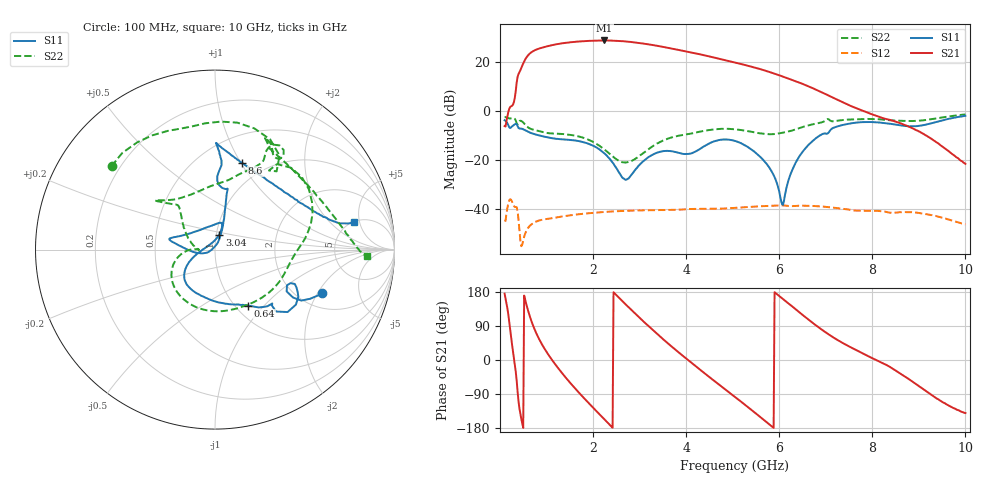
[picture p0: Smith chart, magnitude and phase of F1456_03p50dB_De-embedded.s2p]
! Integrated Device Technology
! Corporate Headquarters
! 6024 Silver Creek Valley Road
! San Jose, CA 95138  USA
! Phone:  1-408-284-8200
! Toll Free:  1-800-223-1366
! Webpage:  http://www.idt.com/
! Timing and RF Division
! 515 Groton Road, Suite 102
! Westford, MA 01886-6024
! Device:  F1456
! Description: 6-bit 0.5 dB Transmit Variable Gain Amplifier
! Frequency:  2100.0 -  2950.00 MHz
! Package:  6x6 mm Thin QFN Plastic Package: 28 pin
! State:  7
! Atten State:  3.5 dB
! Voltage:  +5.00 Volts
! Current:  214.736 mA
! Data:  The device was measured on a the F1455 evaluation board which has
!  individual transmission lines to the RF pins.  Data was collected
!  using a calibrated network analyzer.  The evaluation board was
!  de-embedded using a TRL calibration technique.
!  The reference plane is the edge of the package pin.
!  Pin  1 = CSb
!  Pin  2 = DATA
!  Pin  3 = CLK
!  Pin  4 = RSET
!  Pin  5 = GND
!  Pin  6 = RFIN  = Port 1
!  Pin  7 = GND
!  Pin  8 = NC
!  Pin  9 = NC
!  Pin 10 = NC
!  Pin 11 = NC
!  Pin 12 = NC
!  Pin 13 = NC
!  Pin 14 = /STBY
!  Pin 15 = GND
!  Pin 16 = RFOUT  = Port 2
!  Pin 17 = GND
!  Pin 18 = NC
!  Pin 19 = NC
!  Pin 20 = NC
!  Pin 21 = GND
!  Pin 22 = NC
!  Pin 23 = GND
!  Pin 24 = NC
!  Pin 25 = NC
!  Pin 26 = NC
!  Pin 27 = GND
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# GHz S dB R 50
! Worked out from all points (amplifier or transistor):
!   496 points, 100 MHz to 10 GHz, reference 50 ohm
!   highest |S21| = 28.7 dB at 2.24 GHz (marker M1)
!   |S21| within 3 dB of that: 892.5 MHz to 3.61 GHz (2.717 GHz wide, 121 % of centre)
!   unconditionally stable (mu >= 1): start of sweep to end of sweep
!   at 1.74 GHz: K = 2.25, MAG = 28.8 dB, |S12| = -42.0 dB
!   at 5.06 GHz: K = 3.97, MAG = 20.6 dB, |S12| = -39.5 dB
!   at 10 GHz: K = 131.43, MAG = -11.9 dB, |S12| = -46.2 dB
!   S11 on the Smith chart (normalised r, x): 100 MHz: 2.67, -2.19; 640 MHz: 1.14, -0.82; 3.04 GHz: 1.03, +0.17; 8.6 GHz: 0.78, +1.01; 10 GHz: 5.01, +4.20
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0.1  -3.82 -21.9  -6.19 175.0  -44.59 42.5  -2.61 141.1
0.34  -5.27 -34.2  8.23 -31.4  -39.13 -144.6  -3.94 55.5
0.42  -7.17 -43.2  15.77 -128.8  -48.98 141.3  -4.13 47.2
0.54  -7.86 -52.9  20.84 159.9  -50.06 -169.5  -5.56 10.8
0.64  -8.83 -59.6  23.32 115.9  -46.83 162.6  -7.15 -4.9
0.84  -9.98 -74.1  25.36 55.5  -44.63 114.5  -8.22 -35.6
1.16  -11.25 -100.6  26.90 -6.8  -43.59 70.6  -9.24 -82.8
1.48  -11.80 -121.9  27.86 -56.1  -42.58 43.3  -9.69 -121.7
1.76  -12.59 -136.7  28.32 -94.6  -41.95 24.1  -10.77 -146.6
1.98  -13.98 -146.2  28.55 -123.1  -41.56 10.8  -12.44 -162.2
2.24  -17.24 -158.8  28.66 -156.1  -41.16 -4.1  -15.66 -176.4
2.58  -25.76 165.9  28.44 161.5  -40.80 -22.4  -20.58 179.4
3.04  -21.24 74.1  27.50 106.6  -40.51 -45.5  -17.75 166.2
3.4  -16.90 73.7  26.40 66.3  -40.39 -62.7  -13.11 142.7
4.02  -17.56 112.9  24.08 2.1  -39.98 -89.3  -9.57 130.9
4.52  -13.03 161.0  22.06 -47.1  -39.89 -112.3  -7.74 139.3
5.06  -12.28 169.6  19.63 -98.4  -39.50 -135.1  -7.52 139.2
5.7  -20.97 -167.2  16.36 -161.2  -38.77 -168.5  -9.41 118.9
6.7  -12.58 76.1  9.39 99.8  -38.70 129.7  -5.58 63.1
8.36  -5.20 83.1  -3.60 -16.9  -41.41 56.5  -3.81 62.4
8.6  -5.90 72.7  -5.02 -35.5  -41.27 50.5  -4.04 55.7
10  -2.03 11.4  -21.59 -140.0  -46.22 -25.9  -1.46 -2.5
